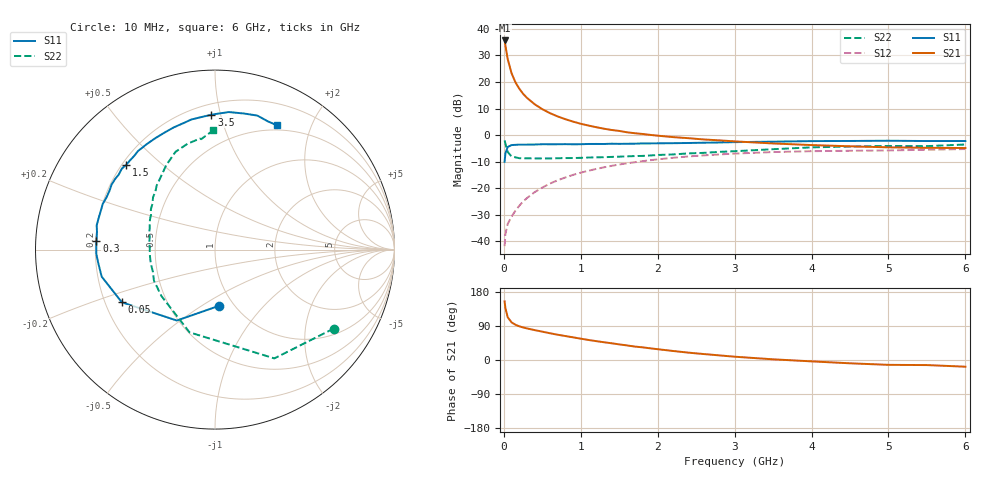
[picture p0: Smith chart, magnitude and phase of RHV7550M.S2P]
! SIEMENS Small Signal Semiconductors
! BFR106
! Si NPN RF Bipolar Junction Transistor in SOT23
! VCE = 0.75 V  IC = 50 mA
! Common Emitter S-Parameters:  August  1996
# GHz  S  MA  R  50
!  f  S11  S21  S12  S22
! GHz  MAG  ANG  MAG  ANG  MAG  ANG  MAG  ANG
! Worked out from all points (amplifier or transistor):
!   36 points, 10 MHz to 6 GHz, reference 50 ohm
!   highest |S21| = 35.6 dB at 10 MHz (marker M1)
!   |S21| within 3 dB of that: start of sweep to 26.82 MHz
!   unconditionally stable (mu >= 1): 173.8 MHz to end of sweep
!   at 250 MHz: K = 1.08, MAG = 18.6 dB, |S12| = -25.0 dB
!   at 1.4 GHz: K = 1.10, MAG = 4.9 dB, |S12| = -11.6 dB
!   at 6 GHz: K = 1.03, MAG = -0.9 dB, |S12| = -5.3 dB
!   S11 on the Smith chart (normalised r, x): 10 MHz: 0.85, -0.59; 50 MHz: 0.27, -0.25; 300 MHz: 0.20, +0.03; 1.5 GHz: 0.22, +0.38; 3.5 GHz: 0.27, +0.94; 6 GHz: 0.44, +1.53
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0.01  0.3145 -86.2  60.53 154.7  0.0081 71.3  0.7948 -33.6
0.02  0.4489 -118.3  49.03 137.3  0.0136 60.2  0.6903 -61.4
0.05  0.5963 -150.5  27.12 112.9  0.0212 51.5  0.4824 -107.1
0.1  0.6491 -166.6  14.65 99.3  0.0291 56.0  0.395 -139.1
0.15  0.6553 -173.8  9.924 93.1  0.0376 60.8  0.3816 -153.0
0.2  0.6613 -177.8  7.515 89.0  0.0466 64.2  0.3671 -160.6
0.25  0.6611 178.7  5.999 85.8  0.056 65.8  0.366 -166.5
0.3  0.662 176.0  5.032 83.4  0.0651 67.7  0.3652 -169.8
0.4  0.6648 171.5  3.815 78.9  0.0842 68.2  0.3642 -175.3
0.5  0.673 168.4  3.075 74.8  0.1029 68.3  0.3635 -179.5
0.6  0.6717 164.4  2.587 70.6  0.1223 67.3  0.3634 177.7
0.7  0.6723 160.6  2.245 66.7  0.141 66.2  0.367 175.0
0.8  0.6752 157.8  1.991 63.2  0.1593 64.6  0.3691 172.2
1.1  0.6805 147.8  1.512 52.9  0.2132 59.6  0.3782 165.8
1.5  0.684 136.4  1.198 41.2  0.2794 52.2  0.3925 157.7
1.7  0.6892 130.8  1.086 35.5  0.3081 48.5  0.4025 153.4
2.2  0.7041 118.2  0.916 23.8  0.3738 39.0  0.4324 143.7
2.8  0.7261 104.1  0.796 12.2  0.4322 28.3  0.4834 132.2
3.5  0.752 91.5  0.696 1.8  0.4793 17.1  0.5427 120.1
4.5  0.7751 78.0  0.615 -8.7  0.5067 3.6  0.6094 104.5
5.5  0.773 67.7  0.576 -13.4  0.5301 -4.4  0.62 97.2
6  0.7734 63.4  0.571 -17.7  0.546 -10.4  0.6647 90.8
